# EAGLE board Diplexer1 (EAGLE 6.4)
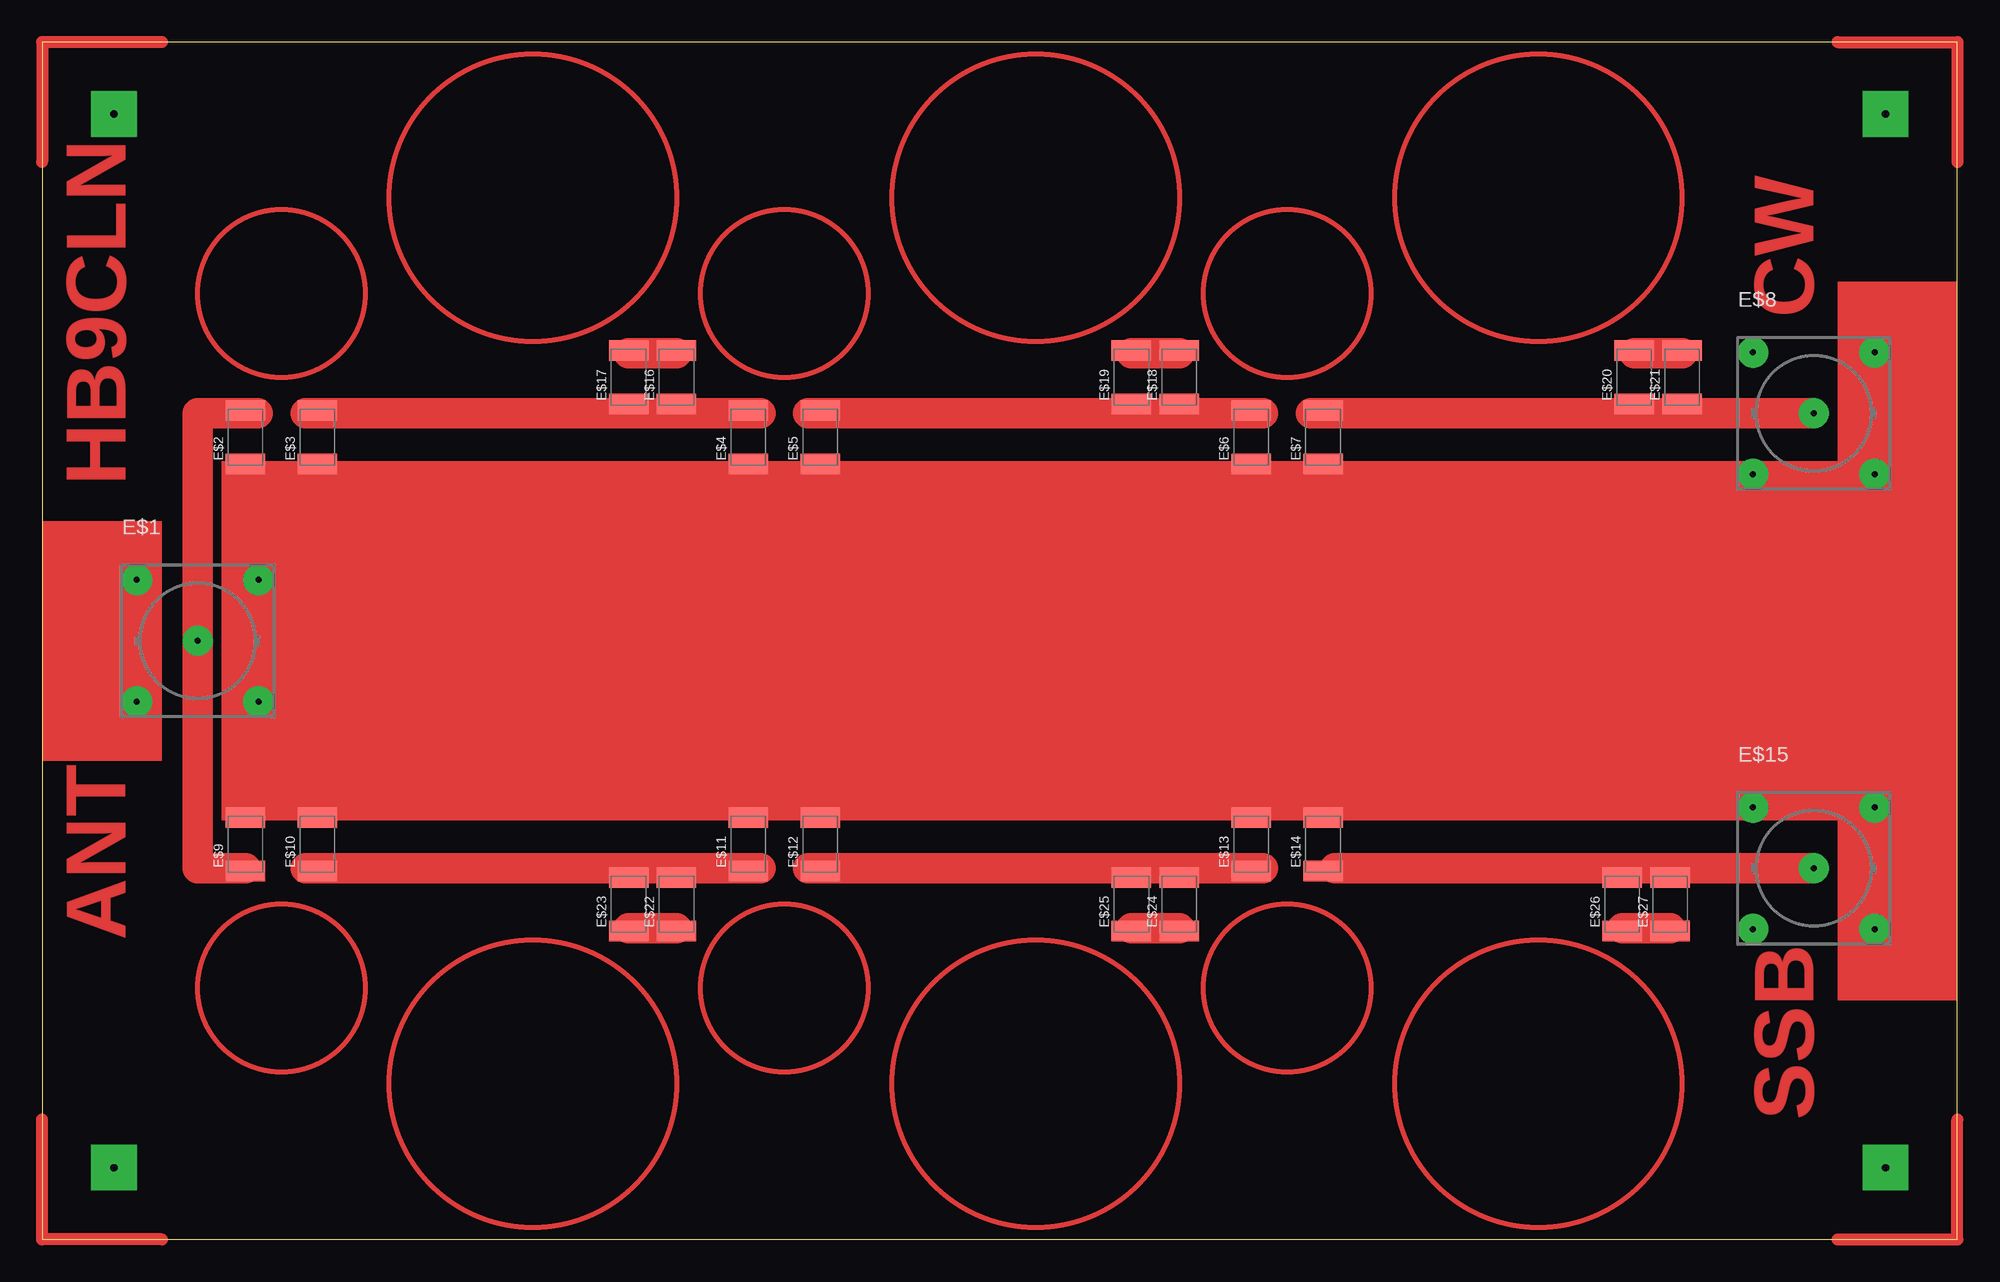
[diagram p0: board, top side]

Size 160 x 100 mm. Coordinates in mm from the lower left corner, seen from the top.
Outline: 0,0 160,0 160,100 0,100 0,0
Copper layers (1*16): Top 0.035mm / dielectric 1.5mm / Bottom 0.035mm
Design rules "default": minimum track width 10mil, minimum drill 24mil, track to track 8mil, track to pad 8mil, pad to pad 8mil, via to via 8mil, smd to smd 8mil, copper to edge 40mil, drill to drill 8mil, minimum pad ring 10mil, minimum via ring 8mil, stop-mask expansion 4mil, vias tented up to drill 0mil, thermal gap 10mil

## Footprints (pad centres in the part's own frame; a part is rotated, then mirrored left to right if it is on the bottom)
BNC-PCB-SQR-HOME = drill 0.5 pad 2.54: 1 0,0; 2 5.08,5.08; 3 -5.08,5.08; 4 -5.08,-5.08; 5 5.08,-5.08
1812 = smd 1.702 x 3.302: 1 -2.235,0; 2 2.235,0

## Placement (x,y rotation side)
E$1  [BNC-PCB-SQR-HOME]  13,50 0 top
E$2  [1812]  17,67 90 top
E$3  [1812]  23,67 90 top
E$4  [1812]  59,67 90 top
E$5  [1812]  65,67 90 top
E$6  [1812]  101,67 90 top
E$7  [1812]  107,67 90 top
E$8  [BNC-PCB-SQR-HOME]  148,69 0 top
E$9  [1812]  17,33 90 top
E$10  [1812]  23,33 90 top
E$11  [1812]  59,33 90 top
E$12  [1812]  65,33 90 top
E$13  [1812]  101,33 90 top
E$14  [1812]  107,33 90 top
E$15  [BNC-PCB-SQR-HOME]  148,31 0 top
E$16  [1812]  53,72 90 top
E$17  [1812]  49,72 90 top
E$18  [1812]  95,72 90 top
E$19  [1812]  91,72 90 top
E$20  [1812]  133,72 90 top
E$21  [1812]  137,72 90 top
E$22  [1812]  53,28 90 top
E$23  [1812]  49,28 90 top
E$24  [1812]  95,28 90 top
E$25  [1812]  91,28 90 top
E$26  [1812]  132,28 90 top
E$27  [1812]  136,28 90 top

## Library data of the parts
E$1 E$8 E$15 = BHE-Connector
E$2-E$7 E$9-E$14 E$16-E$27 = BHE-C

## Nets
S$1: E$1.1

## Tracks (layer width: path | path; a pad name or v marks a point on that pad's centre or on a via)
S$1
  Top 2.54: 18,69 13,69 E$1.1 13,31 17,31
S$2
  Top 2.54: 22,69 60,69
S$3
  Top 2.54: 64,69 102,69
S$4
  Top 2.54: 106,69 148,69
S$5
  Top 2.54: 22,31 60,31
S$6
  Top 2.54: 64,31 102,31
S$7
  Top 2.54: 108,31 148,31
S$8
  Top 2.54: 49,74 53,74
S$9
  Top 2.54: 91,74 95,74
S$10
  Top 2.54: 49,26 53,26
S$11
  Top 2.54: 91,26 95,26
S$12
  Top 2.54: 133,74 137,74
S$13
  Top 2.54: 132,26 136,26
S$14
  Top 1.016: 10,100 0,100 0,90
S$15
  Top 1.016: 10,0 0,0 0,10
S$16  (via drill 0.6 pad 3.81)
  other vias: 6,6 6,94 154,94 154,6
S$17
  Top 1.016: 150,100 160,100 160,90
S$18
  Top 1.016: 150,0 160,0 160,10
(copper drawn outside any net)
  shapes: Top area x3, Top circle x12

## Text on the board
Top: CW | HB9CLN | ANT | SSB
